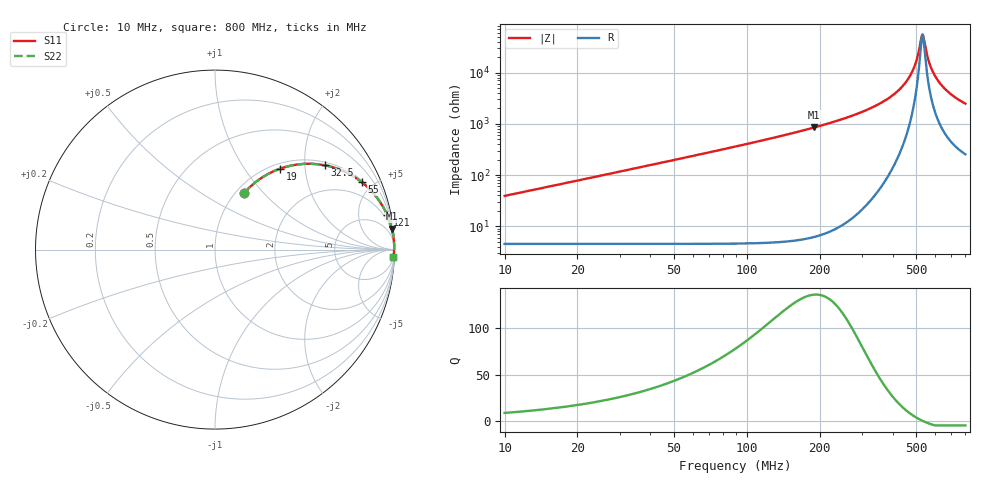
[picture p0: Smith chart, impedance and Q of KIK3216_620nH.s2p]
!version-2
!date-01.2022
!Series
# MHz S RI R 50
!Freq ReS11 ImS11 ReS21 ImS21 ReS12 ImS12 ReS22 ImS22
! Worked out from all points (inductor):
!   528 points, 10 MHz to 800 MHz, reference 50 ohm
!   read as one part in series: L = 620 nH near 13 MHz
!   highest Q = 137 at 190 MHz (marker M1), where L = 711 nH
!   self-resonance near 532 MHz
!   S11 on the Smith chart (normalised r, x): 10 MHz: 1.09, +0.78; 19 MHz: 1.09, +1.48; 32.5 MHz: 1.09, +2.54; 55 MHz: 1.09, +4.33; 121 MHz: 1, +10; 800 MHz: 6, -49
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10  0.1602 0.3131  0.8398 -0.3131  0.8398 -0.3131  0.1602 0.3131
19  0.3634 0.4513  0.6366 -0.4513  0.6366 -0.4513  0.3634 0.4513
32.5  0.6139 0.4693  0.3861 -0.4693  0.3861 -0.4693  0.6139 0.4693
43  0.7344 0.4284  0.2656 -0.4284  0.2656 -0.4284  0.7344 0.4284
55  0.8192 0.3745  0.1808 -0.3745  0.1808 -0.3745  0.8192 0.3745
80.5  0.9082 0.2817  0.0918 -0.2817  0.0918 -0.2817  0.9082 0.2817
121  0.9594 0.1926  0.0406 -0.1926  0.0406 -0.1926  0.9594 0.1926
142  0.9713 0.1628  0.0287 -0.1628  0.0287 -0.1628  0.9713 0.1628
190  0.9855 0.1161  0.0145 -0.1161  0.0145 -0.1161  0.9855 0.1161
274  0.9946 0.0684  0.0054 -0.0684  0.0054 -0.0684  0.9946 0.0684
406  0.9982 0.0264  0.00178 -0.0264  0.00178 -0.0264  0.9982 0.0264
446.5  0.9984 0.017  0.00158 -0.017  0.00158 -0.017  0.9984 0.017
478  0.9984 0.0104  0.00157 -0.0104  0.00157 -0.0104  0.9984 0.0104
505  0.9983 0.00507  0.00165 -0.00507  0.00165 -0.00507  0.9983 0.00507
529  0.9982 0.000608  0.00179 -0.000608  0.00179 -0.000608  0.9982 0.000608
533.5  0.9982 -0.000205  0.00182 0.000205  0.00182 0.000205  0.9982 -0.000205
538  0.9982 -0.00101  0.00185 0.00101  0.00185 0.00101  0.9982 -0.00101
559  0.998 -0.00468  0.00202 0.00468  0.00202 0.00468  0.998 -0.00468
583  0.9978 -0.00872  0.00225 0.00872  0.00225 0.00872  0.9978 -0.00872
619  0.9973 -0.0145  0.00266 0.0145  0.00266 0.0145  0.9973 -0.0145
668.5  0.9966 -0.022  0.00335 0.022  0.00335 0.022  0.9966 -0.022
800  0.9943 -0.0398  0.00573 0.0398  0.00573 0.0398  0.9943 -0.0398
